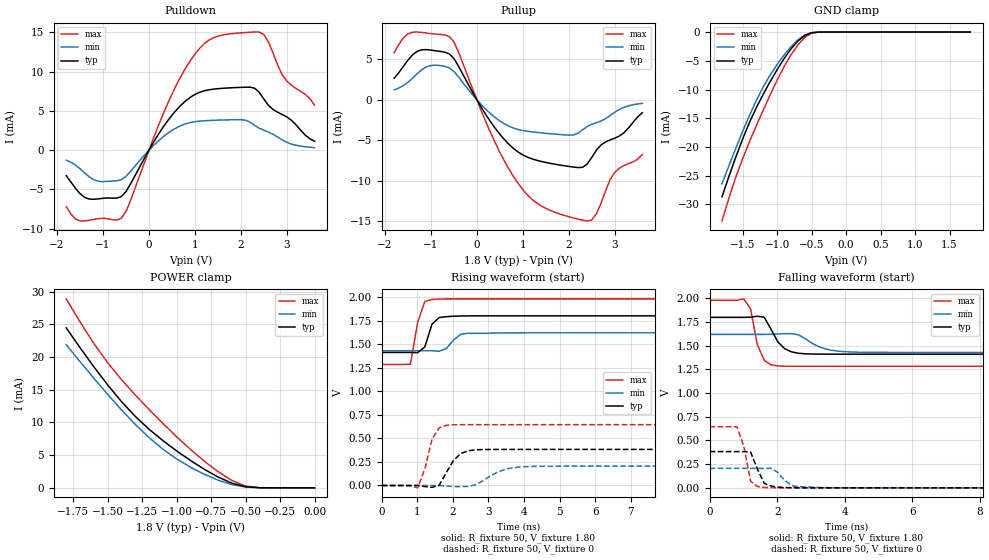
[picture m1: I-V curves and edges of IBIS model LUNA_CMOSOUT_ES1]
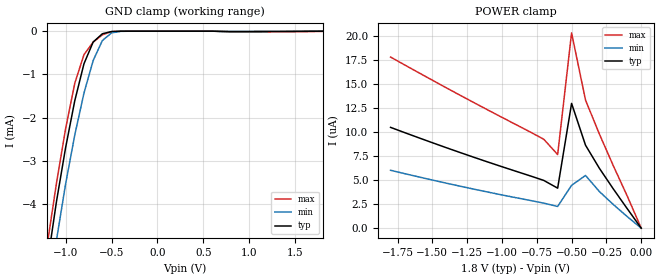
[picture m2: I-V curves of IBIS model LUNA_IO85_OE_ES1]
[IBIS Ver]   3.2
[Comment Char]   |_char
[File name]   sg-8018cx_18v_a.ibs
[File Rev]   1.0
[Date]   2017/09/29 1:38:46
[Source]
[Notes]
[Disclaimer]
This information is for modeling purposes only, and is not guaranteed.
Property of SEIKO EPSON Corp.,
unauthorized reproduction and/or distribution is strictly prohibited.
[Copyright]
Copyright 2017, SEIKO EPSON Corp.
[Component]   SG-8018CA
Si_location Pin
Timing_location Pin
[Manufacturer]   SEIKO EPSON Corp.
| 7050 PKG
| 7050 PKG
[Package]
R_pkg   224m   NA   NA
L_pkg   5.5n   NA   NA
C_pkg   0.144p   NA   NA
[Pin] signal_name   model_name
1   OE   LUNA_IO85_OE_ES1
2   VSS   GND
3   OUT   LUNA_CMOSOUT_ES1
4   VDD   POWER
[Component]   SG-8018CB
Si_location Pin
Timing_location Pin
[Manufacturer]   SEIKO EPSON Corp.
| 5032 PKG
| 5032 PKG
[Package]
R_pkg   200m   NA   NA
L_pkg   2.16n   NA   NA
C_pkg   1.23p   NA   NA
[Pin] signal_name   model_name
1   OE   LUNA_IO85_OE_ES1
2   VSS   GND
3   OUT   LUNA_CMOSOUT_ES1
4   VDD   POWER
[Component]   SG-8018CE
Si_location Pin
Timing_location Pin
[Manufacturer]   SEIKO EPSON Corp.
| 3225 PKG
| 3225 PKG
[Package]
R_pkg   177m   NA   NA
L_pkg   4.5n   NA   NA
C_pkg   0.64p   NA   NA
[Pin] signal_name   model_name
1   OE   LUNA_IO85_OE_ES1
2   VSS   GND
3   OUT   LUNA_CMOSOUT_ES1
4   VDD   POWER
[Component]   SG-8018CG
Si_location Pin
Timing_location Pin
[Manufacturer]   SEIKO EPSON Corp.
| 2520 PKG
| 2520 PKG
[Package]
R_pkg   238m   NA   NA
L_pkg   2.1n   NA   NA
C_pkg   0.38p   NA   NA
[Pin] signal_name   model_name
1   OE   LUNA_IO85_OE_ES1
2   VSS   GND
3   OUT   LUNA_CMOSOUT_ES1
4   VDD   POWER
| Models and submodels in the file (2): LUNA_CMOSOUT_ES1 (3-state), LUNA_IO85_OE_ES1 (Input)
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[Model]   LUNA_CMOSOUT_ES1
Model_type 3-state
Enable Active-High
Polarity Non-Inverting
Vmeas=0.90
C_comp   2.5p   2.0p   3.0p
[Temperature Range] 25   105   -40
[Voltage Range]   1.80   1.62   1.98
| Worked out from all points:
|   slope of the pulldown table from 0 to 0.27 V, typ, clamps not added: 104 ohm
|   slope of the pullup table from 0 to 0.27 V, typ, clamps not added: 109 ohm
|   GND clamp passes 1 mA (typ) near -0.64 V on its own axis
|   POWER clamp passes 1 mA (typ) near -0.63 V on its own axis
|   falling waveform, R_fixture 50, V_fixture 1.80: 20-80 % time 422ps typ, 624ps min, 284ps max; typ from 1.8 V to 1.41 V
|   falling waveform, R_fixture 50, V_fixture 0: 20-80 % time 283ps typ, 348ps min, 243ps max; typ from 0.383 V to 0 V
|   rising waveform, R_fixture 50, V_fixture 1.80: 20-80 % time 216ps typ, 297ps min, 241ps max; typ from 1.41 V to 1.8 V
|   rising waveform, R_fixture 50, V_fixture 0: 20-80 % time 405ps typ, 611ps min, 291ps max; typ from 0 V to 0.383 V
[Pullup]
-1.8V     2.667mA    1.226mA    5.846mA
-1.5V     4.91mA     2.171mA    8.169mA
-1.3V     6.001mA    3.215mA    8.397mA
-1V       6.158mA    4.256mA    8.205mA
-600mV    5.682mA    3.955mA    7.835mA
700mV     -5.525mA   -3.28mA    -8.608mA
1.1V      -7.104mA   -3.895mA   -11.78mA
1.6V      -7.876mA   -4.202mA   -13.71mA
2.3V      -8.358mA   -3.71mA    -14.91mA
2.5V      -7.131mA   -3.031mA   -14.88mA
3V        -4.749mA   -1.534mA   -8.971mA
3.6V      -1.597mA   -440.8uA   -6.77mA
[Pulldown]
-1.8V     -3.251mA   -1.272mA   -7.198mA
-1.6V     -4.852mA   -1.902mA   -8.75mA
-1.4V     -6.009mA   -2.889mA   -9.022mA
-1.1V     -6.198mA   -3.965mA   -8.719mA
-600mV    -5.907mA   -3.747mA   -8.657mA
600mV     5.138mA    2.856mA    8.339mA
1V        7.093mA    3.624mA    12.23mA
1.4V      7.762mA    3.798mA    14.31mA
2.2V      8.014mA    3.556mA    15mA
2.5V      6.487mA    2.536mA    14.69mA
2.9V      4.528mA    1.289mA    9.574mA
3.6V      1.125mA    321.6uA    5.721mA
[GND Clamp]
-1.8V     -28.67mA   -26.41mA   -32.88mA
-1.6V     -21.75mA   -20.22mA   -25.25mA
-1.5V     -18.58mA   -17.27mA   -22mA
-1.4V     -15.69mA   -14.46mA   -19.04mA
-1.2V     -10.77mA   -9.503mA   -13.52mA
-1.1V     -8.591mA   -7.44mA    -10.88mA
-900mV    -4.635mA   -4.001mA   -6.009mA
-700mV    -1.565mA   -1.365mA   -2.263mA
-600mV    -601.2uA   -521.6uA   -925.2uA
-500mV    -121.4uA   -116.4uA   -188.8uA
-400mV    -10.57uA   -14.63uA   -13.06uA
1.8V      99.8pA     105.8nA    71.35pA
[POWER Clamp]
-1.8V     24.46mA    21.89mA    28.9mA
-1.6V     18.52mA    16.76mA    22.08mA
-1.5V     15.75mA    14.3mA     19.15mA
-1.3V     10.93mA    9.714mA    14.21mA
-1.1V     7.236mA    5.92mA     9.861mA
-1V       5.655mA    4.424mA    7.824mA
-900mV    4.191mA    3.162mA    5.894mA
-700mV    1.665mA    1.179mA    2.483mA
-600mV    721.7uA    498.7uA    1.143mA
-500mV    167.2uA    126.9uA    275.1uA
-400mV    16.41uA    18.75uA    19.76uA
0V        99.8pA     596.4pA    86.97pA
[Falling Waveform]
R_fixture=50
V_fixture=1.80
V_fixture_min=1.62
V_fixture_max=1.98
0s        1.8V       1.62V      1.98V
1.01ns    1.8V       1.62V      1.995V
1.212ns   1.802V     1.62V      1.89V
1.414ns   1.812V     1.62V      1.51V
1.616ns   1.802V     1.62V      1.347V
2.02ns    1.541V     1.625V     1.288V
2.626ns   1.421V     1.617V     1.284V
3.434ns   1.412V     1.466V     1.284V
4.242ns   1.411V     1.434V     1.284V
20ns      1.411V     1.43V      1.284V
[Falling Waveform]
R_fixture=50
V_fixture=0
V_fixture_min=0
V_fixture_max=0
0s        382.8mV    205.2mV    645.6mV
808.1ps   382.8mV    205.2mV    644.9mV
1.01ns    382.6mV    205.2mV    444.3mV
1.212ns   378.6mV    205.2mV    71.03mV
1.616ns   46.85mV    205mV      3.979mV
1.818ns   19.71mV    207.3mV    1.243mV
2.02ns    7.936mV    162.5mV    356.9uV
2.424ns   1.591mV    24.05mV    40.22uV
3.232ns   73.06uV    4.312mV    379.3nV
20ns      0V         0V         0V
[Rising Waveform]
R_fixture=50
V_fixture=1.80
V_fixture_min=1.62
V_fixture_max=1.98
0s        1.411V     1.43V      1.284V
808.1ps   1.411V     1.43V      1.287V
1.01ns    1.409V     1.43V      1.73V
1.212ns   1.471V     1.43V      1.952V
1.414ns   1.712V     1.43V      1.974V
1.616ns   1.782V     1.424V     1.979V
1.818ns   1.791V     1.454V     1.98V
2.222ns   1.798V     1.605V     1.98V
2.424ns   1.799V     1.615V     1.98V
20ns      1.8V       1.62V      1.98V
[Rising Waveform]
R_fixture=50
V_fixture=0
V_fixture_min=0
V_fixture_max=0
0s        0V         0V         0V
1.01ns    652.9uV    1.37uV     -24.96mV
1.212ns   -10.91mV   -9.425uV   175.7mV
1.414ns   -19.92mV   119.8uV    491.5mV
1.616ns   3.203mV    389.1uV    611.8mV
1.818ns   137.5mV    -6.559mV   639mV
2.222ns   339mV      -12.45mV   645.5mV
2.828ns   381.3mV    46.13mV    645.6mV
4.242ns   382.8mV    202.4mV    645.6mV
20ns      382.8mV    205.2mV    645.6mV
[Ramp]
R_load=50
dV/dt_r   2.297E-1/3.757E-10   1.231E-1/5.979E-10   3.874E-1/2.579E-10
dV/dt_f   2.331E-1/3.945E-10   1.141E-1/6.153E-10   4.178E-1/2.562E-10
|[End   LUNA_CMOSOUT_ES1
[Model]   LUNA_IO85_OE_ES1
Model_type Input
Enable Active-Low
Polarity Non-Inverting
Vinh=1.39
Vinl=0.48
C_comp   2.5p   2.0p   3.0p
[Temperature Range] 25   105   -40
[Voltage Range]   1.80   1.62   1.98
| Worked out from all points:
|   GND clamp passes 1 mA (typ) near -0.83 V on its own axis
[GND Clamp]
-1.8V     -17.06mA   -17.31mA   -17.53mA
-1.2V     -5.408mA   -6.351mA   -4.953mA
-1.1V     -3.959mA   -4.854mA   -3.533mA
-1V       -2.702mA   -3.543mA   -2.264mA
-900mV    -1.611mA   -2.406mA   -1.207mA
-800mV    -755.6uA   -1.435mA   -543.8uA
-700mV    -251.6uA   -679.9uA   -253.8uA
-600mV    -60.29uA   -218.4uA   -84.58uA
-500mV    -8.175uA   -39.66uA   -10.45uA
-400mV    -667.8nA   -4.047uA   -594nA
800mV     -9.61uA    -4.857uA   -17.73uA
1.8V      72.89pA    2.202uA    -5.276uA
[POWER Clamp]
-1.8V     10.5uA     6.032uA    17.83uA
-1.3V     7.877uA    4.371uA    13.84uA
-700mV    4.977uA    2.609uA    9.265uA
-600mV    4.168uA    2.258uA    7.669uA
-500mV    13uA       4.465uA    20.34uA
-400mV    8.645uA    5.49uA     13.35uA
-300mV    6.229uA    3.813uA    9.792uA
-200mV    4.08uA     2.459uA    6.49uA
-100mV    2.02uA     1.199uA    3.335uA
0V        72.85pA    181.7pA    73.98pA
